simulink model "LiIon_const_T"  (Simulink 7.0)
settings: Solver=ode23tb  StartTime=0.0  StopTime=10000  RelTol=1e-4
undefined symbols (not defined in the file or in its folder): plecs
libraries: plecslib x2

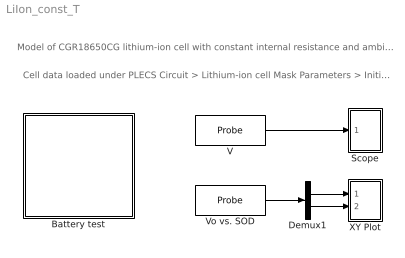
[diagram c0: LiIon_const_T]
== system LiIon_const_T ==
  note: Model of CGR18650CG lithium-ion cell with constant internal resistance and ambient temperature
  note: Cell data loaded under PLECS Circuit > Lithium-ion cell Mask Parameters > Initialization
  Battery test : Subsystem  LoadFcn=plecs('sl', 200);  InitFcn=plecs('sl', 214);  StartFcn=plecs('sl', 208);  StopFcn=plecs('sl', 209);  mask(PlecsCircuit){PLECSData=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}
      mask prompts: PLECSData "PLECS Data (Do not delete or modify!)"
      mask init:
      | % PLACE CUSTOM INITIALIZATIONS ABOVE
      | % DO NOT REMOVE
      | plecs('sl', 215);
      | % DO NOT REMOVE
  Demux1 : Demux  Outputs=2
  Scope : Subsystem  LoadFcn=plecs('sl', 300);  StartFcn=plecs('sl', 308);  StopFcn=plecs('sl', 309);  mask{Settings=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}
      mask init:
      | plecsedit('sl', 315);
  V : plecslib/Probe  SystemSampleTime=-1  tagno=1
  Vo vs. SOD : plecslib/Probe  SystemSampleTime=-1  tagno=3
  XY Plot : Subsystem  LoadFcn=plecs('sl', 317);  StartFcn=plecs('sl', 308);  StopFcn=plecs('sl', 309);  mask{Settings=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}
      mask init:
      | plecs('sl', 315);
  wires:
  Vo vs. SOD/1 -> Demux1/1
  Demux1/1 -> XY Plot/1(1)
  Demux1/2 -> XY Plot/2(2)
  V/1 -> Scope/1(1)

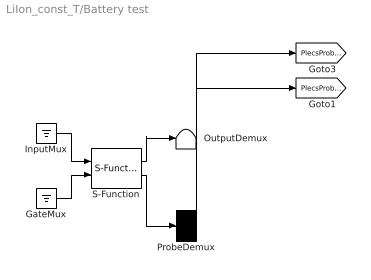
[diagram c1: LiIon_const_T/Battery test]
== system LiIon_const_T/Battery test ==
  " GateMux " : Ground
  " InputMux " : Ground
  " OutputDemux " : Terminator
  " ProbeDemux " : Demux  Outputs=[ 2 1 ]
  " S-Function " : S-Function  FunctionName=plecs
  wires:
  " S-Function "/1 -> " OutputDemux "/1
  " InputMux "/1 -> " S-Function "/1
  " GateMux "/1 -> " S-Function "/2
  " S-Function "/2 -> " ProbeDemux "/1
  " ProbeDemux "/1 -> [PlecsProbe3]
  " ProbeDemux "/2 -> [PlecsProbe1]

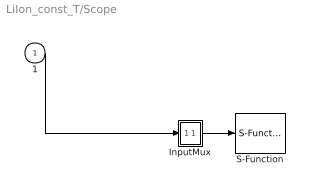
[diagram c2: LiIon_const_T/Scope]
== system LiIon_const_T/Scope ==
  1 : Inport  OutDataType=sfix(16)  OutScaling=2^0
  " InputMux " : Subsystem
  " S-Function " : S-Function  FunctionName=plecs
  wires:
  " InputMux "/1(Out) -> " S-Function "/1
  1/1 -> " InputMux "/1(In1)

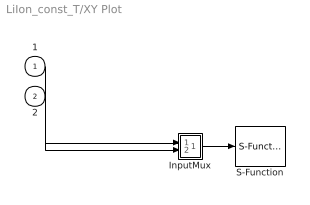
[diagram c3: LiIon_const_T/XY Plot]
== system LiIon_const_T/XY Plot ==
  1 : Inport
  2 : Inport  Port=2
  " InputMux " : Subsystem
  " S-Function " : S-Function  FunctionName=plecs
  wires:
  " InputMux "/1(Out) -> " S-Function "/1
  1/1 -> " InputMux "/2(In2)
  2/1 -> " InputMux "/1(In1)

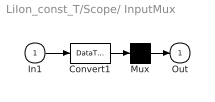
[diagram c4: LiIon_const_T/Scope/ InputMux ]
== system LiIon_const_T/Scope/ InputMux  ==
  In1 : Inport  OutDataType=sfix(16)  OutScaling=2^0
  Convert1 : DataTypeConversion  OutDataType=sfix(16)  OutScaling=2^0
  Mux : Mux  Inputs=1
  Out : Outport  OutDataType=sfix(16)  OutScaling=2^0
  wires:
  Mux/1 -> Out/1
  In1/1 -> Convert1/1
  Convert1/1 -> Mux/1

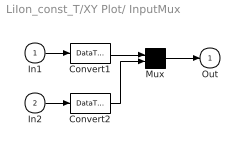
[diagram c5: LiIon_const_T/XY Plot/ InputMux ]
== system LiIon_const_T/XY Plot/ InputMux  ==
  In1 : Inport
  In2 : Inport  Port=2
  Convert1 : DataTypeConversion
  Convert2 : DataTypeConversion
  Mux : Mux  Inputs=2
  Out : Outport
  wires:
  Mux/1 -> Out/1
  In1/1 -> Convert1/1
  Convert1/1 -> Mux/1
  In2/1 -> Convert2/1
  Convert2/1 -> Mux/2
